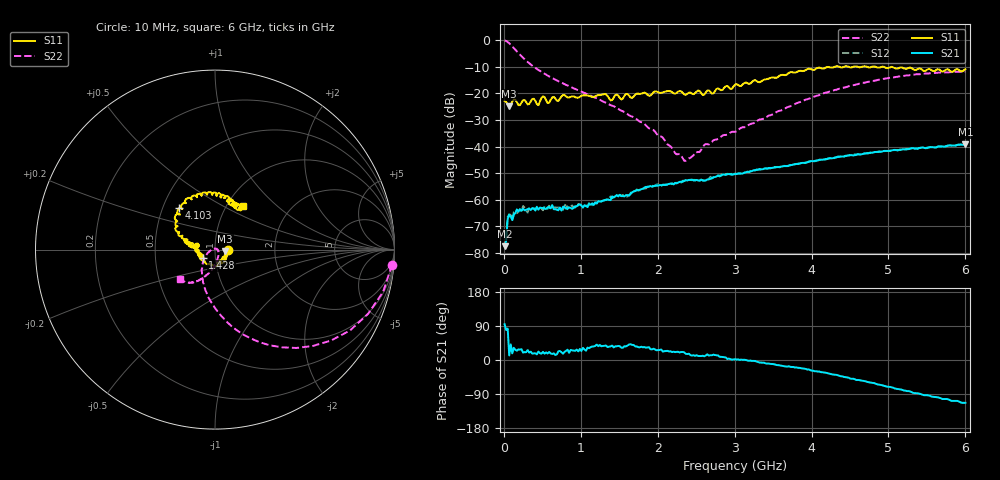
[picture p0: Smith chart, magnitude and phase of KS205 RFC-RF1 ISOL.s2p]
!Agilent	"Technologies,E5071B,JP1KK00126,A.08.11"
!Date:	Wed	Mar	27	12:08:32	2013
!Data	&	Calibration	Information:
!Freq	S11:SOLT2(ON)	S21:SOLT2(ON)	S12:SOLT2(ON)	S22:SOLT2(ON)
#	Hz	S	dB	R	50
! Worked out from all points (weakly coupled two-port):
!   301 points, 10 MHz to 6 GHz, reference 50 ohm
!   highest |S21| = -39.10 dB at 6 GHz (marker M1); lowest = -77.4 dB at 10 MHz (marker M2)
!   lowest |S11| = -24.8 dB at 69.9 MHz (marker M3), VSWR 1.12, Z = 56 - j0.934 ohm
!   |S11| at or under -10 dB: start of sweep to 4.3 GHz; 4.832 GHz to 4.915 GHz (83.19 MHz wide, 1.71 % of centre); 4.942 GHz to end of sweep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
!   |S22| runs from -45.3 to -0.1 dB; largest |S21 - S12| = 0.00026
!   S11 on the Smith chart (normalised r, x): 10 MHz: 1.16, -0.01; 1.428 GHz: 0.87, -0.08; 4.103 GHz: 0.61, +0.31; 6 GHz: 1.19, +0.62
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1e7  -22.80 -1.8  -77.40 94.2  -74.20 120.0  -0.09 -4.9
2.996667e7  -23.20 -8.9  -75.40 79.2  -73.00 60.6  -0.30 -14.1
4.993333e7  -24.20 -12.1  -67.20 83.0  -66.40 95.2  -0.68 -22.8
6.99e7  -24.80 -8.3  -65.70 12.0  -65.40 16.9  -1.14 -30.9
1.098333e8  -23.00 -4.3  -67.60 17.4  -67.30 21.4  -2.33 -44.6
1.298e8  -22.30 -11.8  -65.60 32.2  -64.60 36.6  -2.96 -50.4
1.897e8  -24.40 -24.9  -64.30 28.0  -64.50 25.8  -4.86 -64.4
3.294667e8  -24.00 -30.5  -63.20 19.7  -63.00 21.2  -8.64 -84.8
3.893667e8  -22.00 -45.4  -63.30 17.5  -63.20 18.6  -9.98 -91.0
4.492667e8  -24.40 -44.9  -63.70 22.3  -63.20 17.8  -11.20 -96.7
5.091667e8  -21.10 -54.5  -63.10 21.5  -63.90 19.8  -12.20 -101.0
5.690667e8  -23.60 -68.3  -62.80 17.1  -63.40 16.7  -13.30 -106.0
1.0283e9  -20.70 -118.0  -62.90 32.0  -62.30 24.8  -19.60 -131.0
1.427633e9  -21.60 -146.0  -59.00 33.2  -59.10 34.9  -24.80 -149.0
2.006667e9  -19.60 178.0  -54.70 26.3  -54.10 24.2  -35.90 175.0
2.366067e9  -20.50 168.0  -52.60 16.3  -52.60 18.9  -45.30 91.9
2.625633e9  -19.60 175.0  -52.70 12.0  -52.60 11.1  -39.00 26.4
3.005e9  -16.70 172.0  -50.30 2.2  -50.10 2.8  -34.40 -18.5
4.0233e9  -11.20 135.0  -45.50 -28.4  -45.40 -28.6  -21.30 -90.5
4.103167e9  -10.30 131.0  -44.90 -30.6  -45.00 -30.8  -20.60 -93.1
5.001667e9  -10.40 88.7  -41.60 -70.8  -41.60 -70.9  -14.20 -118.0
6e9  -10.90 57.4  -39.10 -113.0  -39.20 -113.0  -11.80 -140.0
